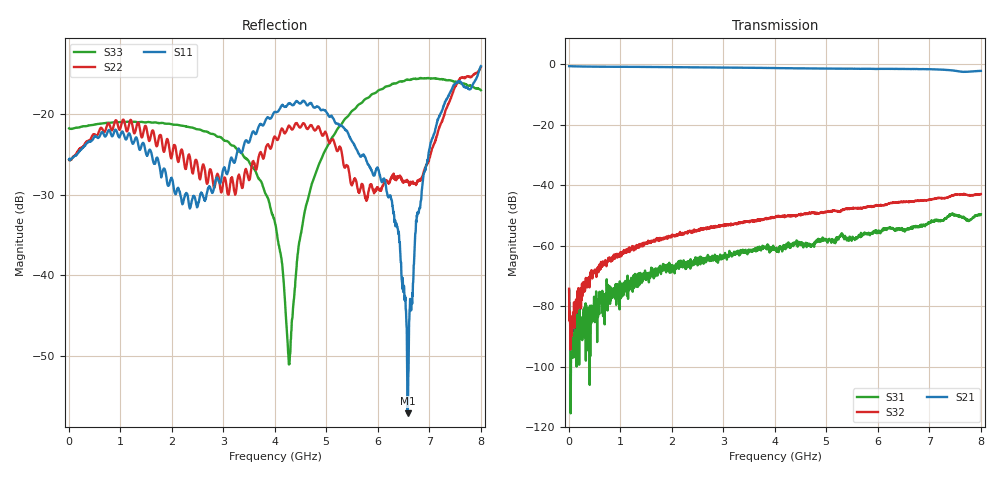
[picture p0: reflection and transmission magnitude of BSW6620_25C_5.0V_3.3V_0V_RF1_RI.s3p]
! Product: BSW6620
! Temp: 25C
! VDD: 5.000
! Control_Hi: 3.300
! Control_Lo: 0.000
! Logic State: RF1
! Port 1: RFC
! Port 2: RF1
! Port 3: RF2
! V1 = 5.00
! V2 = 0.00
! V3 = 0.00
! V4 = 0.00
# Hz S  RI  R 50
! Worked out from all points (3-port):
!   1601 points, 5 MHz to 8.005 GHz, reference 50 ohm
!   strongest paths, dB at 5 MHz, 2.005 GHz, 4.005 GHz, 6.005 GHz, 8.005 GHz:
!     S21: -0.6, -0.9, -1.2, -1.5, -2.2
!     S32: -74.2, -56.9, -50.5, -46.7, -42.9
!     S31: -74.6, -67.6, -61.0, -55.5, -49.6
!   lowest |S11| = -57.2 dB at 6.58 GHz (marker M1), VSWR 1.00, Z = 50.1 - j0.124 ohm
!   |S11| at or under -10 dB: start of sweep to end of sweep
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5000000  0.0524 0.000258  0.9327 -0.0129  0.000147 -0.000109
         0.9328 -0.0132  0.0521 -0.000217  0.000159 -8.26e-05
         0.000146 -0.000115  0.000155 -0.000116  0.0819 -0.00079
7.15e8  0.0554 -0.0479  0.0645 -0.9099  0.000101 4.84e-05
        0.0639 -0.9104  0.0571 -0.0559  0.000534 0.000131
        0.000125 3.67e-05  0.000494 0.00013  0.0618 -0.0632
1.405e9  -0.0267 -0.0569  -0.8886 -0.179  0.000131 -0.000162
         -0.8891 -0.1794  -0.0365 -0.0634  0.000523 -0.000879
         0.000235 -0.000188  0.000457 -0.000974  -0.0118 -0.089
2.2e9  -0.0108 0.0261  -0.099 0.8898  -0.000362 -0.000407
       -0.0988 0.8905  -0.0322 0.0503  -0.00127 -0.000908
       -0.000302 -0.00042  -0.00129 -0.000925  -0.0807 -0.0266
2.96e9  0.0348 -0.018  0.8811 0.0867  -0.000561 0.000255
        0.8815 0.0866  0.033 -0.0014  -0.00151 0.00148
        -0.000544 0.000283  -0.00155 0.00153  -0.0528 0.0487
4.005e9  -0.1038 0.00249  -0.4268 -0.7546  0.000863 0.000389
         -0.428 -0.7549  -0.0715 0.013  0.00274 0.00127
         0.000796 0.000395  0.00267 0.00131  0.0101 0.0187
4.285e9  -0.0935 0.0709  -0.7682 -0.3936  0.000909 0.000156
         -0.7681 -0.3932  -0.0565 0.0631  0.00316 -0.000371
         0.000935 0.000128  0.00311 -0.000277  -0.00145 0.0024
5.26e9  0.0576 0.0628  -0.00944 0.8441  -2.44e-05 -0.00143
        -0.00846 0.8439  0.0534 0.0327  -0.000954 -0.00354
        -3.88e-05 -0.00144  -0.000987 -0.00359  -0.0689 0.0485
6.58e9  0.000614 -0.00124  0.2979 -0.7843  -0.00119 0.0015
        0.2967 -0.7826  0.0263 -0.0278  -0.00235 0.00471
        -0.00127 0.00148  -0.00238 0.0048  0.0931 0.1355
8.005e9  0.1968 0.0321  -0.3659 0.6883  0.00254 -0.00221
         -0.365 0.6889  0.173 0.0935  0.00545 -0.00464
         0.0025 -0.00219  0.00537 -0.00473  0.1019 -0.0981
